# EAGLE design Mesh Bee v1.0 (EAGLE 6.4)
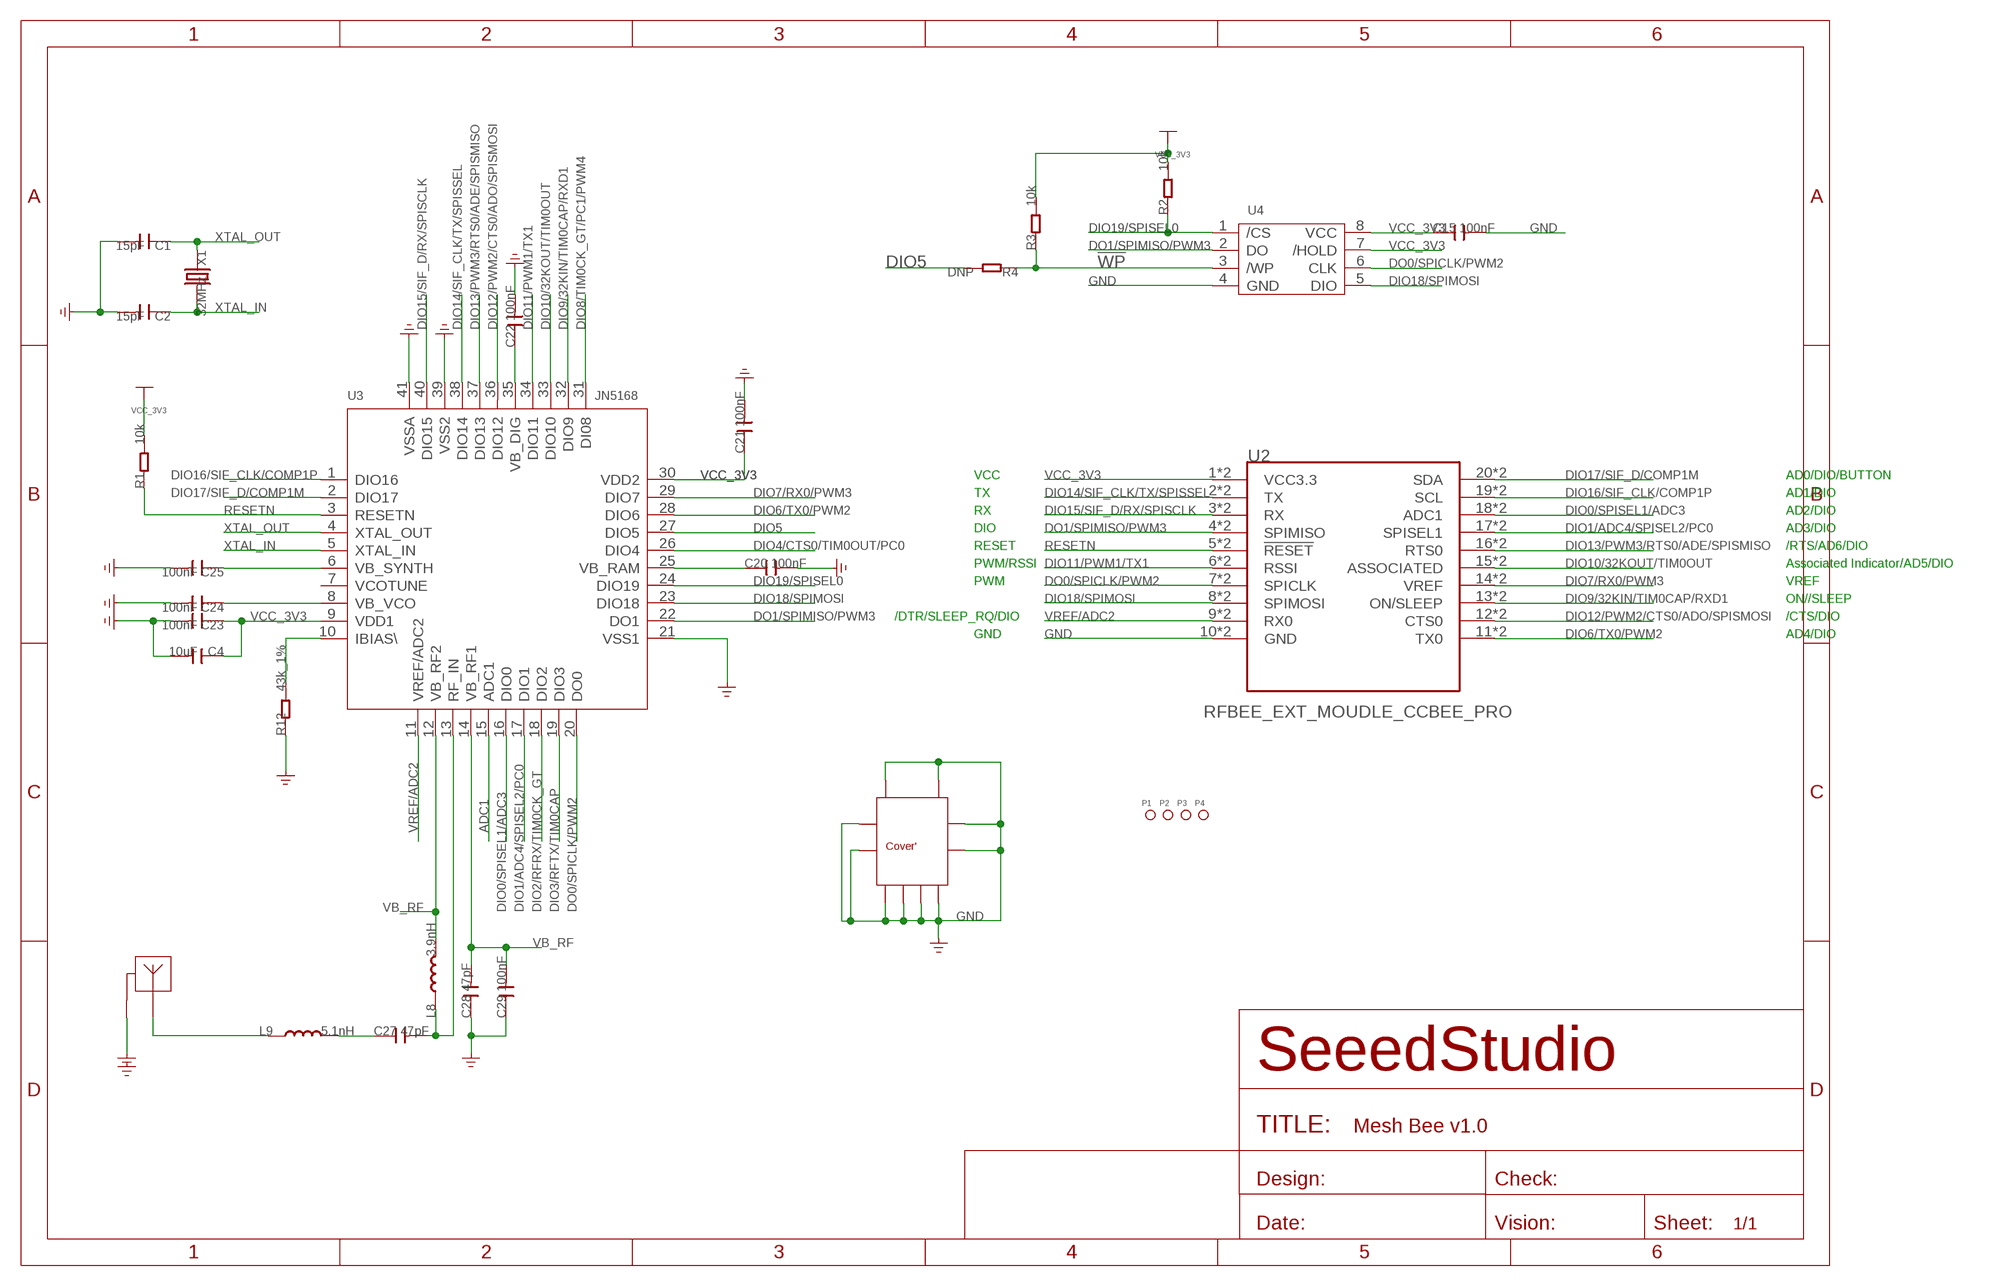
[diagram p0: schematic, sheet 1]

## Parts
ANT1  2.4G-ANT  [2.4G-ANT]
C1  15pF  C-0402  [C0402]
C2  15pF  C-0402  [C0402]
C4  10uF  C-0603  [C0603]
C15  100nF  C-0402  [C0402]
C20  100nF  C-0402  [C0402]
C21  100nF  C-0402  [C0402]
C22  100nF  C-0402  [C0402]
C23  100nF  C-0402  [C0402]
C24  100nF  C-0402  [C0402]
C25  100nF  C-0402  [C0402]
C27  47pF  C-0402  [C0402]
C28  47pF  C-0402  [C0402]
C29  100nF  C-0402  [C0402]
L8  3.9nH  L'0402'  [L0402]
L9  5.1nH  L'0402'  [L0402]
P1  PAD-MARK  [ROUND-MARK-1.0]
P2  PAD-MARK  [ROUND-MARK-1.0]
P3  PAD-MARK  [ROUND-MARK-1.0]
P4  PAD-MARK  [ROUND-MARK-1.0]
R1  10k  R-0402  [R0402]
R2  10k  R-0402  [R0402]
R3  10k  R-0402  [R0402]
R4  DNP  R-0402  [R0402]
R12  43k_1%  R-0402  [R0402]
U1  TEMPLATE_SHIELDING-COVER  [TEMPLATE_SHIELDING-COVER-20.6X18.5]
U2  RFBEE_EXT_MOUDLE_CCBEE_PRO  [RFBEE_EXT_MOUDLE_CCBEE-PRO]
U3  JN5168  [HVQFN40]
U4  W25X80  [WSON8]
X1  32MHz  CRYSTAL'3225'  [4P-SMD-3.2X2.5]

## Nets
!WP: R3.1 R4.1 U4.3(/WP)
ADC1: U3.15(ADC1)
DIO0/SPISEL1/ADC3: U2.18(ADC1) U2.P18(ADC1) U3.16(DIO0)
DIO1/ADC4/SPISEL2/PC0: U2.17(SPISEL1) U2.P17(SPISEL1) U3.17(DIO1)
DIO2/RFRX/TIM0CK_GT: U3.18(DIO2)
DIO3/RFTX/TIM0CAP: U3.19(DIO3)
DIO4/CTS0/TIM0OUT/PC0: U3.26(DIO4)
DIO5: R4.2 U3.27(DIO5)
DIO6/TX0/PWM2: U2.11(TX0) U2.P11(TX0) U3.28(DIO6)
DIO7/RX0/PWM3: U2.14(VREF) U2.P14(VREF) U3.29(DIO7)
DIO8/TIM0CK_GT/PC1/PWM4: U3.31(DI08)
DIO9/32KIN/TIM0CAP/RXD1: U2.13(ON/SLEEP) U2.P13(ON/SLEEP) U3.32(DIO9)
DIO10/32KOUT/TIM0OUT: U2.15(ASSOCIATED) U2.P15(ASSOCIATED) U3.33(DIO10)
DIO11/PWM1/TX1: U2.6(RSSI) U2.P6(RSSI) U3.34(DIO11)
DIO12/PWM2/CTS0/ADO/SPISMOSI: U2.12(CTS0) U2.P12(CTS0) U3.36(DIO12)
DIO13/PWM3/RTS0/ADE/SPISMISO: U2.16(RTS0) U2.P16(RTS0) U3.37(DIO13)
DIO14/SIF_CLK/TX/SPISSEL: U2.2(TX) U2.P2(TX) U3.38(DIO14)
DIO15/SIF_D/RX/SPISCLK: U2.3(RX) U2.P3(RX) U3.40(DIO15)
DIO16/SIF_CLK/COMP1P: U2.19(SCL) U2.P19(SCL) U3.1(DIO16)
DIO17/SIF_D/COMP1M: U2.20(SDA) U2.P20(SDA) U3.2(DIO17)
DIO18/SPIMOSI: U2.8(SPIMOSI) U2.P8(SPIMOSI) U3.23(DIO18) U4.5(DIO)
DIO19/SPISEL0: R2.1 U3.24(DIO19) U4.1(/CS)
DO0/SPICLK/PWM2: U2.7(SPICLK) U2.P7(SPICLK) U3.20(DO0) U4.6(CLK)
DO1/SPIMISO/PWM3: U2.4(SPIMISO) U2.P4(SPIMISO) U3.22(DO1) U4.2(DO)
GND: ANT1.1 C1.2 C2.2 C4.2 C15.2 C20.2 C21.2 C22.2 C23.2 C24.2 C25.2 C28.1 C29.1 R12.1 U1.P$1 U1.P$2 U1.P$3 U1.P$4 U1.P$5 U1.P$6 U1.P$7 U1.P$8 U1.P$9 U1.P$10 U2.10(GND) U2.P10(GND) U3.21(VSS1) U3.39(VSS2) U3.41(VSSA) U4.4(GND)
N$1: ANT1.2 L9.1
N$19: C20.1 U3.25(VB_RAM)
N$23: C22.1 U3.35(VB_DIG)
N$24: C25.1 U3.6(VB_SYNTH)
N$25: C24.1 U3.8(VB_VCO)
N$32: R12.2 U3.10(IBIAS\)
N$36: C27.2 L8.1 U3.13(RF_IN)
N$38: C27.1 L9.2
RESETN: R1.1 U2.5(!RESET) U2.P5(!RESET) U3.3(RESETN)
VB_RF: C28.2 C29.2 L8.2 U3.12(VB_RF2) U3.14(VB_RF1)
VCC_3V3: C4.1 C15.1 C21.1 C23.1 R1.2 R2.2 R3.2 U2.1(VCC3.3) U2.P1(VCC3.3) U3.9(VDD1) U3.30(VDD2) U4.7(/HOLD) U4.8(VCC)
VREF/ADC2: U2.9(RX0) U2.P9(RX0) U3.11(VREF/ADC2)
XTAL_IN: C2.1 U3.5(XTAL_IN) X1.4
XTAL_OUT: C1.1 U3.4(XTAL_OUT) X1.2
Unconnected: U3.7(VCOTUNE)

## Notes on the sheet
- VCC | AD0/DIO/BUTTON
- TX | AD1/DIO
- RX | AD2/DIO
- DIO | AD3/DIO
- RESET | /RTS/AD6/DIO
- PWM/RSSI | Associated Indicator/AD5/DIO
- PWM | VREF
- ON//SLEEP
- /DTR/SLEEP_RQ/DIO | /CTS/DIO
- GND | AD4/DIO

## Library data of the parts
ANT1 = template (quxiaohui quxiaohui 的冲突副本 2013-09-17):2.4G-ANT
C1 C2 C4 C15 C20-C25 C27-C29 = Discrete:C*: Ceramic Capacitors
L8 L9 = Discrete:L*
P1-P4 = Discrete:PAD-MARK; PARTNO: DNP
R1-R4 R12 = Discrete:R*
U1 = RFBee_-_REVA:TEMPLATE_SHIELDING-COVER
U2 = RFBee_-_REVA:RFBEE_EXT_MOUDLE_CCBEE
U3 = IC:JN5168: IEEE802.15.4 Wireless Microcontroller
U4 = template:W25X80: 1M-BIT,2M-BIT,4M-BIT AND 8M-BIT SERIAL FLASH MEMORY WITH 4KB SECTORS AND DUAL OUTPUT SPI
X1 = Discrete:CRYSTAL*: CRYSTAL

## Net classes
0 default: width 0.152 mm, drill 0.305 mm, clearance 0.152 mm

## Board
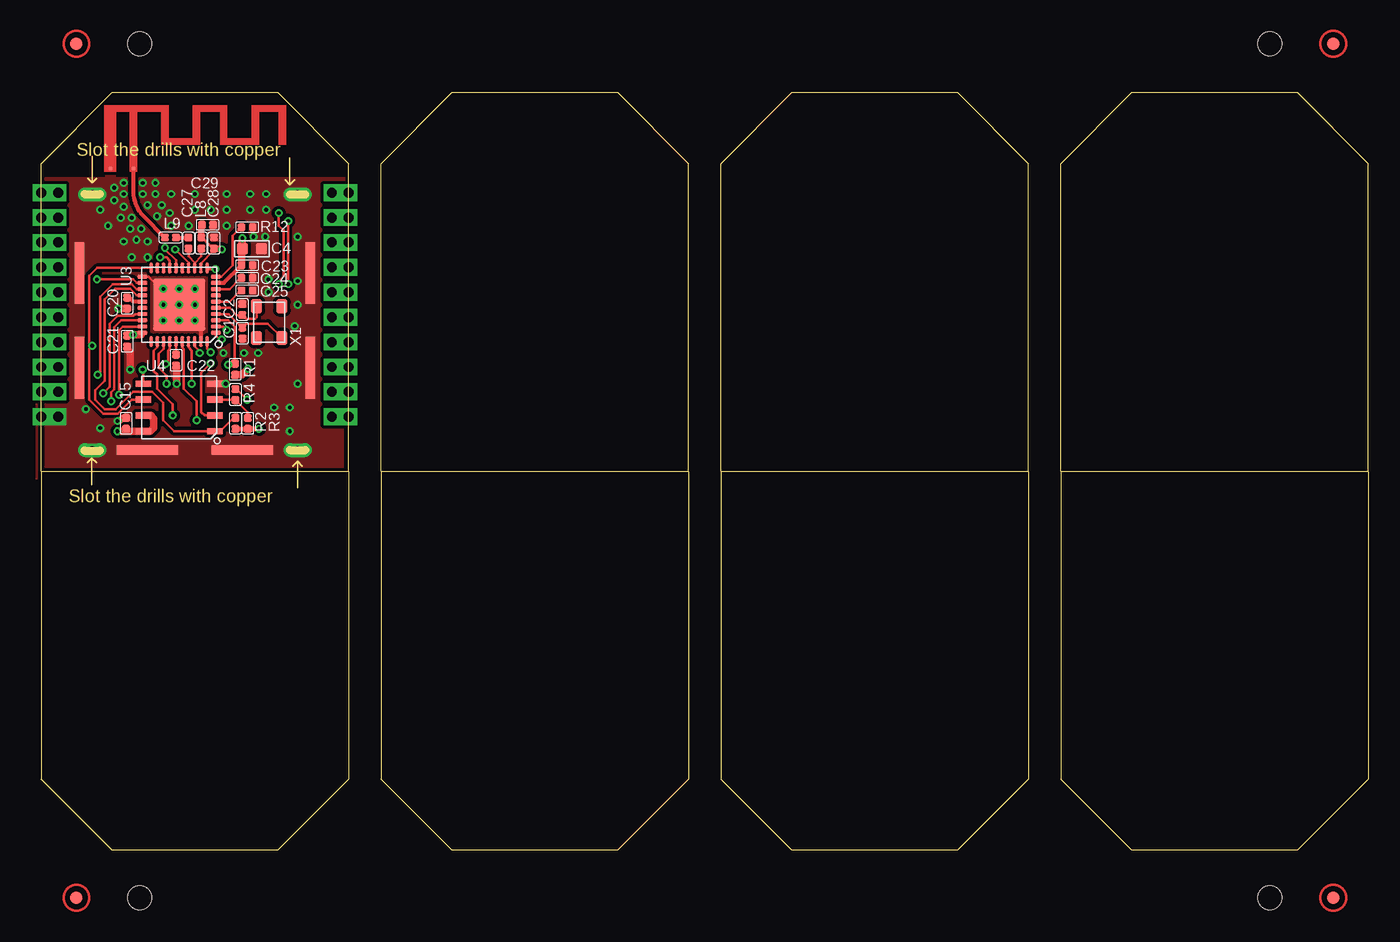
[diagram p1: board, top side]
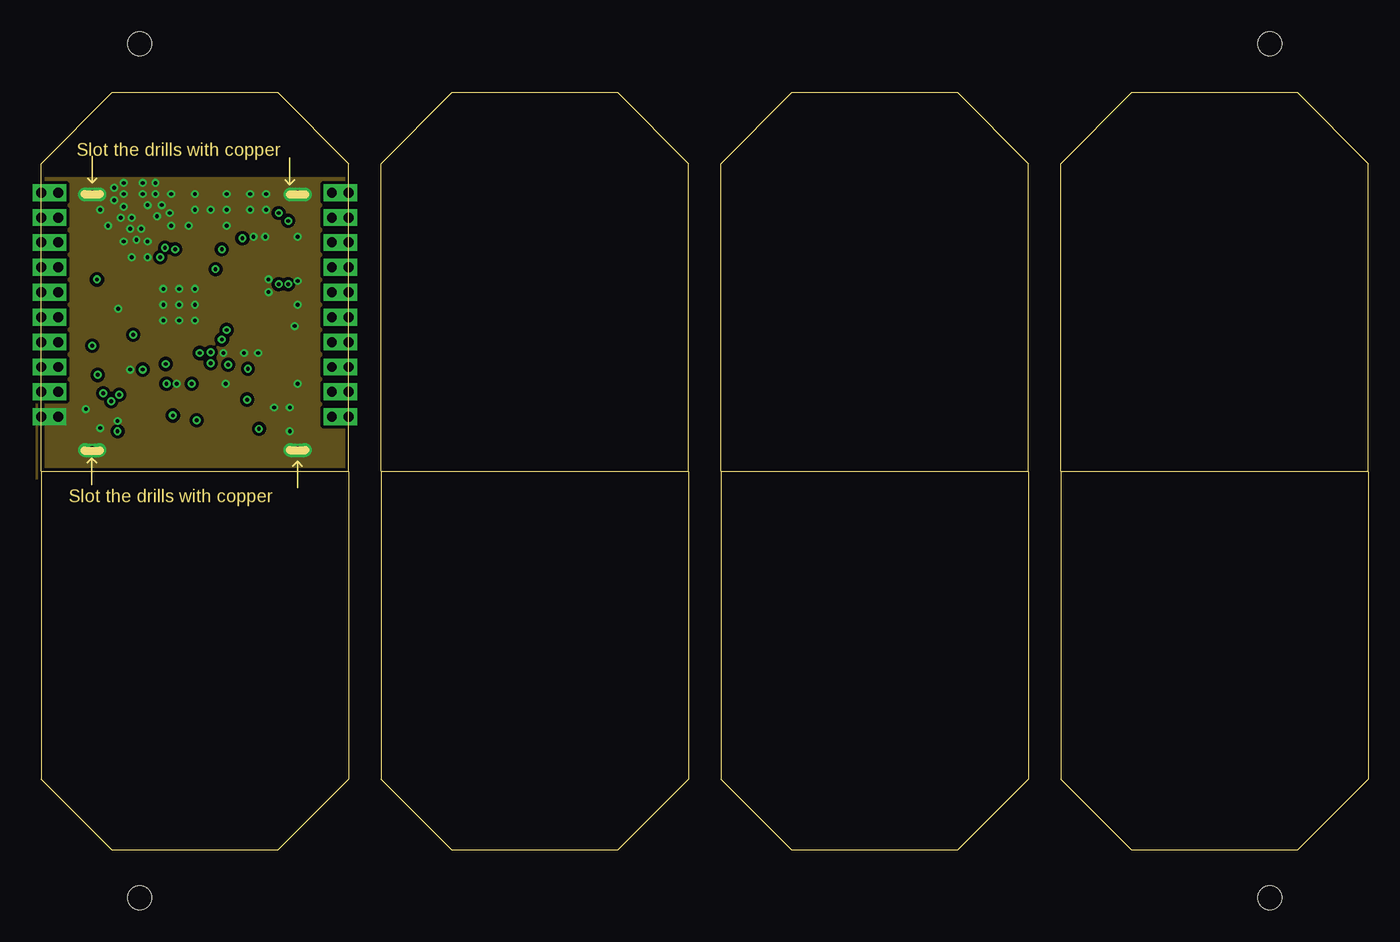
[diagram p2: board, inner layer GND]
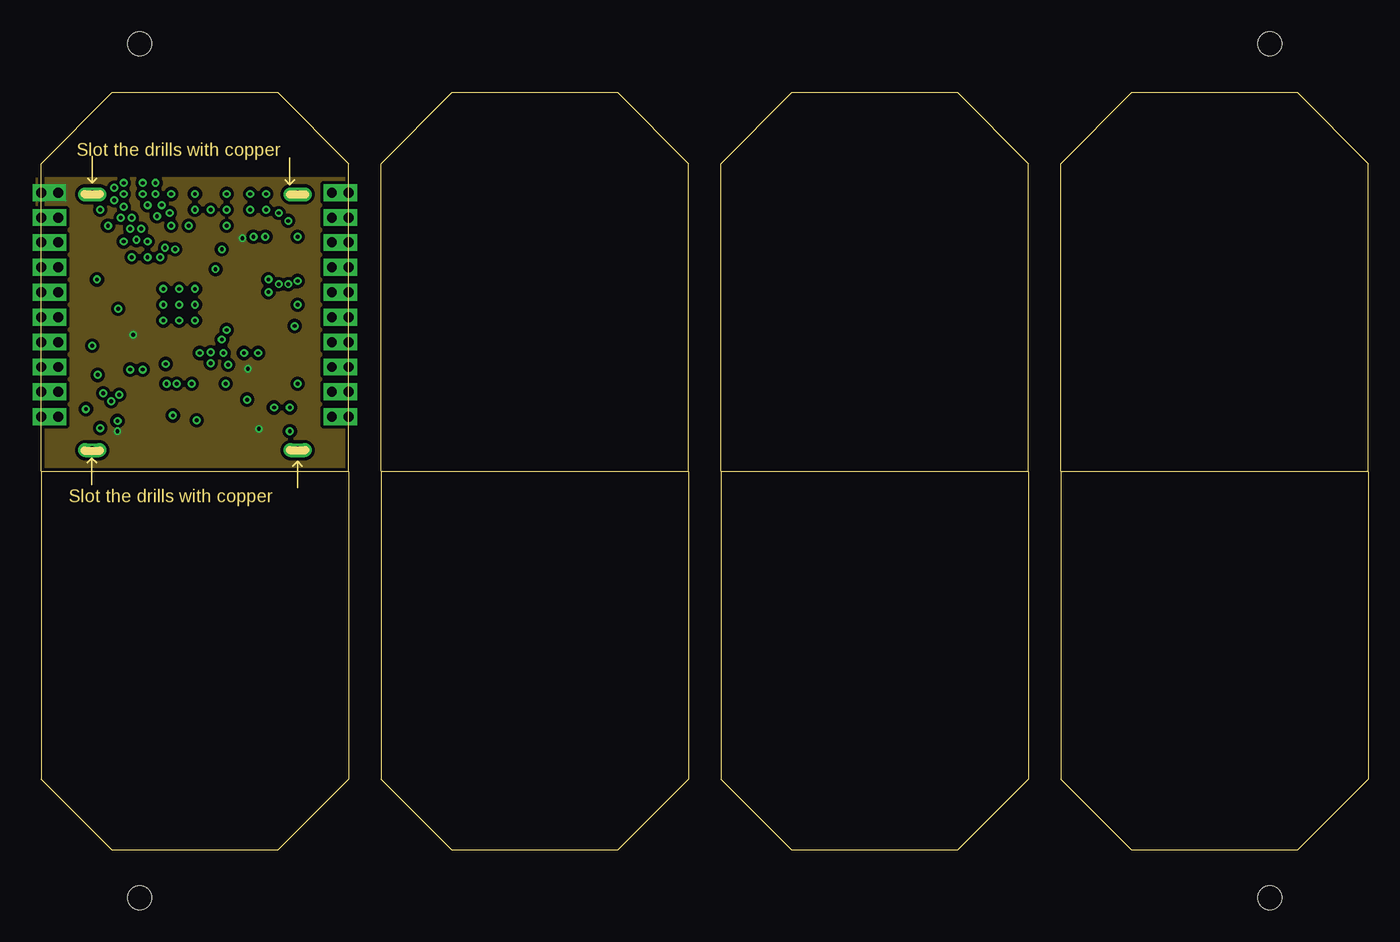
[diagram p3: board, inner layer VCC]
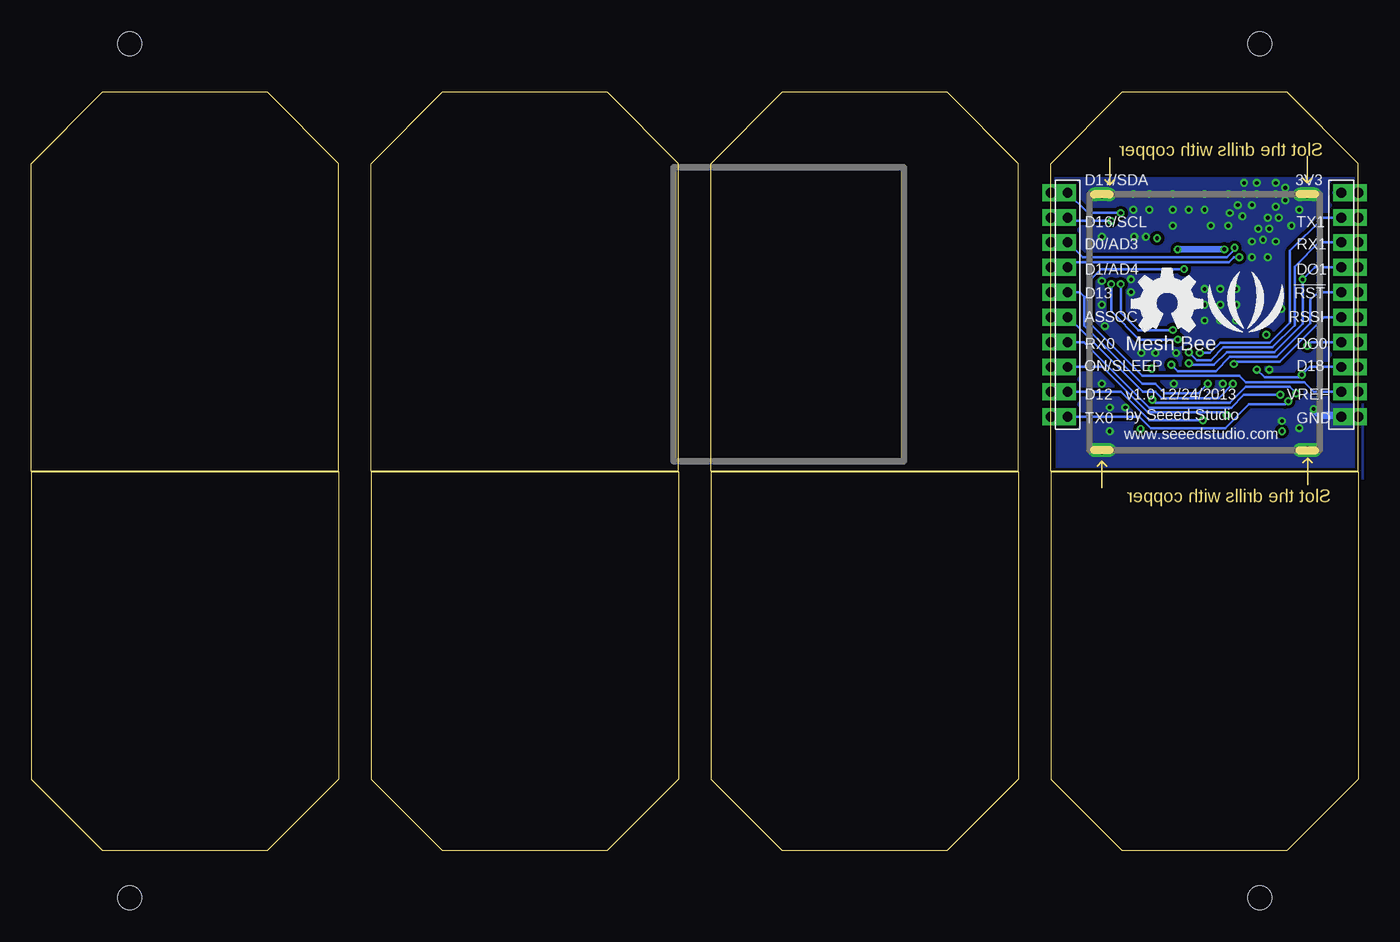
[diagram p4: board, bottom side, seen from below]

Size 106.61 x 60.87 mm. Coordinates in mm from the lower left corner, seen from the top.
Outline: 5.71,60.87 18.98,60.87 24.7,55.16 24.7,30.45 0,30.45 0,55.16 5.71,60.87
Outline: 18.98,0 5.71,0 0,5.71 0,30.43 24.7,30.43 24.7,5.71 18.98,0
Outline: 33.02,60.87 46.29,60.87 52.01,55.16 52.01,30.45 27.3,30.45 27.3,55.16 33.02,60.87
Outline: 46.29,0 33.02,0 27.3,5.71 27.3,30.43 52.01,30.43 52.01,5.71 46.29,0
Outline: 60.33,60.87 73.59,60.87 79.31,55.16 79.31,30.45 54.61,30.45 54.61,55.16 60.33,60.87
Outline: 73.59,0 60.33,0 54.61,5.71 54.61,30.43 79.31,30.43 79.31,5.71 73.59,0
Outline: 87.63,60.87 100.9,60.87 106.61,55.16 106.61,30.45 81.91,30.45 81.91,55.16 87.63,60.87
Outline: 100.9,0 87.63,0 81.91,5.71 81.91,30.43 106.61,30.43 106.61,5.71 100.9,0
Copper layers (1*2+15*16): Top 0.035mm / dielectric 0.2mm / GND 0.0175mm / dielectric 0.4mm / VCC 0.0175mm / dielectric 0.2mm / Bottom 0.035mm
Design rules "SeeedStudio_rule_no_angle_090911 *": minimum track width 6mil, minimum drill 12mil, track to track 6mil, track to pad 6mil, pad to pad 6mil, via to via 6mil, smd to smd 0mil, copper to edge 10mil, drill to drill 10mil, minimum pad ring 10mil, minimum via ring 6mil, stop-mask expansion 2mil, vias tented up to drill 100mil, thermal gap 10mil
Holes 1.91 mm at 7.9,64.78 98.71,64.78 7.9,-3.8 98.71,-3.8
tKeepout: area -4,47.9 to 30.3,61.1; area 29.4,47.3 to 63.7,60.5
tRestrict: area 24.6,29 to 24.6,34.2
bRestrict: area 24.6,29 to 24.6,34.2

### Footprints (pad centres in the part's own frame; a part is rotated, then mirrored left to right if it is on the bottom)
2.4G-ANT = smd 0.305 x 0.305: 1 0.457,0.254; 2 2.286,0.254
C0402 = smd 0.635 x 0.635: 1 -0.445,0; 2 0.445,0
C0603 = smd 0.889 x 0.889: 1 -0.762,0; 2 0.762,0
L0402 = smd 0.635 x 0.635: 1 -0.445,0; 2 0.445,0
ROUND-MARK-1.0 = smd 1.016 x 1.016: P$1 0,0
R0402 = smd 0.635 x 0.635: 1 -0.445,0; 2 0.445,0
TEMPLATE_SHIELDING-COVER-20.6X18.5 = drill 0.635 long: P$1 -8.255,-11.684; P$2 8.255,8.865; P$3 -8.255,8.865; P$4 8.255,-11.684 | smd 0.762 x 4.953: P$5 -9.271,2.54; P$6 -9.271,-5.055; P$7 9.271,2.54; P$8 9.271,-5.055 | smd 4.953 x 0.762: P$9 -3.81,-11.684; P$10 3.81,-11.684
RFBEE_EXT_MOUDLE_CCBEE-PRO = drill 0.8 pad 1.35 square: 1 -11,9; 2 -11,7; 3 -11,5; 4 -11,3; 5 -11,1; 6 -11,-1; 7 -11,-3; 8 -11,-5; 9 -11,-7; 10 -11,-9; 11 11,-9; 12 11,-7; 13 11,-5; 14 11,-3; 15 11,-1; 16 11,1; 17 11,3; 18 11,5; 19 11,7; 20 11,9; P1 -12.35,9; P2 -12.35,7; P3 -12.35,5; P4 -12.35,3; P5 -12.35,1; P6 -12.35,-1; P7 -12.35,-3; P8 -12.35,-5; P9 -12.35,-7; P10 -12.35,-9; P11 12.35,-9; P12 12.35,-7; P13 12.35,-5; P14 12.35,-3; P15 12.35,-1; P16 12.35,1; P17 12.35,3; P18 12.35,5; P19 12.35,7; P20 12.35,9
HVQFN40 = smd 0.8 x 0.3: 1 -2.95,2.25; 2 -2.95,1.75; 3 -2.95,1.25; 4 -2.95,0.75; 5 -2.95,0.25; 6 -2.95,-0.25; 7 -2.95,-0.75; 8 -2.95,-1.25; 9 -2.95,-1.75; 10 -2.95,-2.25; 21 2.95,-2.25; 22 2.95,-1.75; 23 2.95,-1.25; 24 2.95,-0.75; 25 2.95,-0.25; 26 2.95,0.25; 27 2.95,0.75; 28 2.95,1.25; 29 2.95,1.75; 30 2.95,2.25 | smd 0.3 x 0.8: 11 -2.25,-2.95; 12 -1.75,-2.95; 13 -1.25,-2.95; 14 -0.75,-2.95; 15 -0.25,-2.95; 16 0.25,-2.95; 17 0.75,-2.95; 18 1.25,-2.95; 19 1.75,-2.95; 20 2.25,-2.95; 31 2.25,2.95; 32 1.75,2.95; 33 1.25,2.95; 34 0.75,2.95; 35 0.25,2.95; 36 -0.25,2.95; 37 -0.75,2.95; 38 -1.25,2.95; 39 -1.75,2.95; 40 -2.25,2.95 | smd 4.2 x 4.2: 41 0,0
WSON8 = smd 0.5 x 1.25: 1 -1.905,-2.875; 2 -0.635,-2.875; 3 0.635,-2.875; 4 1.905,-2.875; 5 1.905,2.875; 6 0.635,2.875; 7 -0.635,2.875; 8 -1.905,2.875
4P-SMD-3.2X2.5 = smd 1.143 x 0.889: 1 -1.27,1.016; 2 -1.27,-1.016; 3 1.27,-1.016; 4 1.27,1.016

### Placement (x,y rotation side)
ANT1  5.11,54.49 0 top
C1  16.16,41.54 270 top
C2  16.16,43.44 90 top
C4  16.92,48.32 0 top
C15  6.81,34.3 90 top
C20  6.89,43.95 270 top
C21  6.89,40.9 270 top
C22  10.83,39.38 270 top
C23  16.54,47 0 top
C24  16.54,45.98 0 top
C25  16.54,44.96 0 top
C27  11.84,48.77 270 top
C28  13.87,48.77 270 top
C29  13.37,50.24 180 top
L8  12.86,48.77 90 top
L9  10.38,49.22 0 top
P1  not placed on the board
P2  not placed on the board
P3  not placed on the board
P4  not placed on the board
R1  15.58,38.64 270 top
R2  15.6,34.3 270 top
R3  16.59,34.3 270 top
R4  15.6,36.61 90 top
R12  16.54,50.04 180 top
U1  12.35,43.82 0 top
U2  12.35,43.82 0 top
U3  11.08,43.82 180 top
U4  11.08,35.57 90 top
U$16  [OSHW_FILLX200_NOTEXT]  18.19,41.66 0 bottom
U$17  [LOGO_SILK]  9.05,43.31 0 bottom
X1  18.32,42.42 90 top

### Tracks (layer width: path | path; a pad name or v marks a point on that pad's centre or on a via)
!WP
  Top 0.203: R3.1 16.59,35.17 R4.1 15.56,36.2 U4.3
DIO0/SPISEL1/ADC3  (via drill 0.3)
  Top 0.203: U3.16 10.83,47.37 9.94,48.27 v9.94,48.39
  Bottom 0.203: U2.18 23.32,48.82 22.13,47.63 10.57,47.63 9.94,48.27 v9.94,48.39
  Bottom 0.813: U2.18 U2.P18
DIO1/ADC4/SPISEL2/PC0  (via drill 0.3)
  Top 0.203: U3.17 10.33,47.37 10.06,47.63 v9.56,47.63
  Bottom 0.203: v9.56,47.63 10,47.63 10.38,47.25 22.92,47.25 U2.17
  Bottom 0.813: U2.17 U2.P17
DIO5  (via drill 0.3 pad 0.64)
  Top 0.203: U3.27 7.54,43.07 7.4,42.93 6.13,42.93 5.49,42.3 5.49,37.22 v4.98,36.71 | R4.2 15.69,37.05 v16.54,36.2
  Bottom 0.203: v4.98,36.71 5.49,37.22 9.05,37.22 10.32,35.95 16.29,35.95 v16.54,36.2
DIO6/TX0/PWM2  (via drill 0.3 pad 0.64)
  Top 0.203: U3.28 6.43,42.57 5.87,42.02 5.87,37.03 5.62,36.77 v5.62,36.07
  Bottom 0.203: v5.62,36.07 5.87,35.82 8.79,35.82 10.7,33.92 16.67,33.92 17.57,34.82 U2.11
  Bottom 0.813: U2.11 U2.P11
DIO7/RX0/PWM3  (via drill 0.3 pad 0.64)
  Top 0.203: U3.29 6.54,42.07 6.25,41.79 v6.25,36.58
  Bottom 0.203: v6.25,36.58 9.18,36.58 10.19,35.57 16.8,35.57 22.05,40.82 U2.14
  Bottom 0.813: U2.14 U2.P14
DIO9/32KIN/TIM0CAP/RXD1  (via drill 0.3 pad 0.64)
  Top 0.203: U3.32 9.33,40.42 9.05,40.14 9.05,38.49 9.3,38.23 9.3,37.09 10.57,35.82 v10.57,34.93
  Bottom 0.203: v10.57,34.93 10.83,35.19 16.92,35.19 20.56,38.82 U2.13
  Bottom 0.813: U2.13 U2.P13
DIO10/32KOUT/TIM0OUT  (via drill 0.3 pad 0.64)
  Top 0.203: U3.33 9.83,40.29 9.43,39.88 9.43,38.74 10.06,38.11 v10.06,37.47
  Bottom 0.203: U2.15 23.29,42.82 17.3,36.84 16.29,36.84 15.78,36.33 11.21,36.33 v10.06,37.47
  Bottom 0.813: U2.15 U2.P15
DIO11/PWM1/TX1  (via drill 0.3 pad 0.64)
  Top 0.203: U3.34 10.33,40.28 10.19,40.14 10.19,39.25 v10,39.06
  Bottom 0.203: U2.6 2.75,42.82 6.32,39.25 9.81,39.25 v10,39.06
  Bottom 0.813: U2.6 U2.P6
DIO12/PWM2/CTS0/ADO/SPISMOSI  (via drill 0.3 pad 0.64)
  Top 0.203: U3.36 11.33,40.4 11.46,40.27 11.46,37.09 12.48,36.07 v12.48,34.55
  Bottom 0.203: v12.48,34.55 16.8,34.55 19.07,36.82 U2.12
  Bottom 0.813: U2.12 U2.P12
DIO13/PWM3/RTS0/ADE/SPISMISO  (via drill 0.3 pad 0.64)
  Top 0.203: U3.37 11.83,40.4 12.1,40.14 v12.1,37.47
  Bottom 0.203: U2.16 22.37,44.82 22,44.46 22,42.14 17.33,37.47 16.29,37.47 15.52,36.71 12.86,36.71 v12.1,37.47
  Bottom 0.813: U2.16 U2.P16
DIO14/SIF_CLK/TX/SPISSEL  (via drill 0.3 pad 0.64)
  Top 0.203: U3.38 12.35,40.85 12.35,40.46 12.73,40.07 v12.73,39.95
  Bottom 0.203: U2.2 2.81,50.82 5.49,48.14 5.49,42.39 7.11,40.77 11.08,40.77 11.9,39.95 v12.73,39.95
  Bottom 0.813: U2.2 U2.P2
DIO15/SIF_D/RX/SPISCLK  (via drill 0.3 pad 0.64)
  Top 0.203: v13.62,40.01 13.33,40.3 U3.40
  Bottom 0.203: U2.3 3.16,48.82 5.11,46.87 5.11,42.18 6.9,40.39 10.83,40.39 11.84,39.38 12.98,39.38 v13.62,40.01
  Bottom 0.813: U2.3 U2.P3
DIO16/SIF_CLK/COMP1P  (via drill 0.3, 0.3 pad 0.64)
  Top 0.203: U3.1 14.03,41.38 14.38,41.03 v14.51,41.03 | v19.84,45.47 v19.84,50.55
  Bottom 0.203: v14.51,41.03 17.58,41.03 19.84,43.29 v19.84,45.47 | v19.84,50.55 23.08,50.55 U2.19
  Bottom 0.813: U2.19 U2.P19
DIO17/SIF_D/COMP1M  (via drill 0.3, 0.3 pad 0.64)
  Top 0.203: v19.08,51.19 19.08,50.17 19.46,49.79 19.46,46.11 19.08,45.73 v19.08,45.47 | U3.2 14.61,42.07 v14.89,41.79
  Bottom 0.203: v19.08,51.19 21.72,51.19 U2.20 | v19.08,45.47 19.08,43.19 17.68,41.79 v14.89,41.79
  Bottom 0.813: U2.20 U2.P20
DIO18/SPIMOSI  (via drill 0.3 pad 0.64)
  Top 0.203: U4.5 8.21,38.57 v8.16,38.61 | U3.23 7.67,45.07 7.27,45.47 5.75,45.47 4.73,44.46 4.73,38.38 v4.54,38.19
  Bottom 0.203: v8.16,38.61 7.52,37.98 4.75,37.98 v4.54,38.19 3.9,38.82 U2.8
  Bottom 0.813: U2.8 U2.P8
DIO19/SPISEL0
  Top 0.203: U3.24 7.66,44.57 7.14,45.09 5.92,45.09 5.11,44.28 5.11,37.73 4.35,36.96 4.35,36.2 5.11,35.44 6,35.44 7.4,36.84 8.92,36.84 9.81,35.95 9.81,34.55 10.7,33.66 U4.1 14.38,33.66 15.4,34.68 15.54,34.68 R2.1
DO0/SPICLK/PWM2  (via drill 0.3 pad 0.64)
  Top 0.203: U3.20 4.5,46.77 3.86,46.13 3.86,40.75 v4.09,40.52 3.86,40.28 3.86,36.19 4.98,35.06 6.13,35.06 7.27,36.2 U4.6
  Bottom 0.203: U2.7 3.79,40.82 v4.09,40.52
  Bottom 0.813: U2.7 U2.P7
DO1/SPIMISO/PWM3  (via drill 0.3 pad 0.64)
  Top 0.203: 8.29,45.6 8.16,45.6 U3.22 7.68,45.57 7.4,45.85 v4.48,45.85 | U4.2 13.11,34.93 12.85,35.2 12.85,38.35 v13.62,39.12
  Bottom 0.203: U2.4 3.51,46.82 v4.48,45.85 4.48,42.28 6.74,40.01 10.57,40.01 11.59,39 13.49,39 v13.62,39.12
  Bottom 0.813: U2.4 U2.P4
GND  (via drill 0.3 pad 0.64)
  Top 0.203: U3.21 8.64,46.07 9.56,45.15 9.75,45.15 v9.81,45.09
  Top 0.305: 13.87,50.17 C29.1
  Top 0.33: 10.19,44.58 10.32,44.58 U3.41 12.83,42.07 U3.39
  Top 0.508: 6.25,34.49 v6.13,34.49 6.32,34.49 6.63,34.8 6.89,34.8
  Top 0.61: C20.2 v6.19,43.5 | v10.89,37.47 10.89,38.87 C22.2 | C21.2 6.89,40.27 7.14,40.01 v7.14,38.61 | U4.4 v14.83,37.47
  Bottom 0.61: 1.46,34.93 3.08,34.93 v3.59,35.44
  Bottom 0.813: 1.46,34.93 U2.10 U2.P10
  other vias: 8.54,47.63 18.26,44.84 18.26,45.85 18,49.28 20.61,43.82 20.35,42.11 14.64,39.95 16.29,39.95 17.43,39.95 7.27,47.63 8.54,48.9 8.03,49.92 7.27,50.81 6.63,51.7 6.63,52.71 6.63,53.6 8.16,53.6 8.16,52.71 8.54,51.82 9.3,50.93 10.45,50.17 11.84,50.17 9.68,51.82 12.35,51.44 14.89,51.44 14.89,50.17 13.62,51.44 9.18,53.6 9.18,52.71 12.35,52.71 14.89,52.71 16.8,52.71 16.8,51.44 18.06,52.71 18.06,51.44 20.61,45.73 20.61,49.28 17.05,49.28 6.38,50.81 7.14,49.92 5.87,53.22 7.65,49.03 19.97,33.66 19.97,35.57 18.7,35.57 20.61,37.47 4.73,33.92 11.08,43.82 12.35,45.09 11.08,45.09 9.81,43.82 12.35,43.82 12.35,42.55 11.08,42.55 9.81,42.55 10.32,51.19 10.45,52.71 5.87,52.2 6.63,48.9 5.36,50.17 4.73,51.44
  pour Top (isolate 0.254, no thermals): 5.92,54.62 5.19,54.62 5.19,53.88 5.92,53.88
  pour GND (isolate 0.254, no thermals): -0.35,53.98 25.05,53.98 25.05,29.85 -0.35,29.85
  pour Bottom (isolate 0.254, no thermals): -0.35,53.98 25.05,53.98 25.05,29.85 -0.35,29.85
  pour Top (isolate 0.254, no thermals): -0.35,53.98 25.05,53.98 25.05,29.85 -0.35,29.85
N$1
  Top 0.33: ANT1.2 7.4,52.88 arc45 8.19,50.97 L9.1
N$19
  Top 0.305: U3.25 7.4,44.07 7.14,44.33 6.95,44.33 C20.1
N$23
  Top 0.203: U3.35 C22.1
N$24
  Top 0.203: U3.6 15.14,44.07 16.03,44.96 C25.1
N$25
  Top 0.203: U3.8 15.12,45.07 16.03,45.98 C24.1
N$32
  Top 0.203: U3.10 14.47,46.07 15.4,47 15.4,49.35 R12.2
N$36
  Top 0.203: U3.13 12.33,47.17 | 12.33,47.17 12.86,47.69 L8.1 | 12.33,47.17 12.33,47.21 11.84,47.69 C27.2
N$38
  Top 0.33: L9.2 C27.1
RESETN  (via drill 0.3 pad 0.64)
  Top 0.203: U3.3 15,42.57 15.52,42.04 15.52,39.14 R1.1 15.49,39 v15.02,39
  Bottom 0.203: v15.02,39 14.51,38.49 11.46,38.49 10.32,39.63 6.53,39.63 3.84,42.32 3.84,44.2 3.22,44.82 U2.5
  Bottom 0.813: U2.5 U2.P5
VB_RF  (via drill 0.3)
  Top 0.203: U3.12 12.83,47.16 13.81,48.14 13.81,48.27 | U3.14 11.83,47.2 v10.76,48.27 | 13.81,48.27 C28.2 | 13.81,48.27 13.75,48.27
  Top 0.254: L8.2 12.92,49.22 13.75,48.39 13.75,48.27
  Top 0.305: 12.86,50.17 C29.2
  Top 0.508: 12.86,50.17 L8.2 | C28.2 14.45,48.33 v14.51,48.27
  Bottom 0.508: v10.76,48.27 v14.51,48.27
VCC_3V3  (via drill 0.3, 0.3 pad 0.64)
  Top 0.305: U3.9 14.67,45.57 C23.1 | 8.03,41.41 8.03,41.47 U3.30
  Top 0.406: v17.49,33.85 R3.2 R2.2
  Top 0.61: v16.16,49.16 C4.1 16.1,48.25 C23.1 | C21.1 6.95,41.41 v7.4,41.41 8.03,41.41 | 7,33.66 U4.8 8.76,33.66 9.05,33.95 9.05,34.68 8.79,34.93 U4.7 | 7,33.66 C15.1 | v6.13,33.66 7,33.66 | R1.2 16.12,38.2 v16.61,38.68
  Bottom 0.61: U2.1 1.78,52.82
  Bottom 0.813: U2.1 U2.P1
  pour VCC (isolate 0.254, no thermals): -0.35,53.98 25.05,53.98 25.05,29.85 -0.35,29.85
VREF/ADC2  (via drill 0.3)
  Top 0.203: v14,46.68 13.42,46.68 U3.11
  Bottom 0.203: U2.9 3.57,36.82 4.35,37.6 9.05,37.6 9.56,38.11 17.35,38.11 21.49,42.25 21.49,45.85 20.67,46.68 v14,46.68
  Bottom 0.813: U2.9 U2.P9
XTAL_IN
  Top 0.203: X1.4 17.3,42.81 17.18,42.68 16.48,42.68 C2.1 15.71,43 15.14,43.57 U3.5
XTAL_OUT
  Top 0.203: U3.4 15.07,43.07 C1.1 | 16.1,41.92 C1.1 | X1.2 18.19,42.3 16.48,42.3 C1.1

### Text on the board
bPlace: 3V3 | D17/SDA | TX1 | D16/SCL | RX1 | D0/AD3 | DO1 | D1/AD4 | !RST | D13 | RSSI | ASSOC | DO0 | Mesh Bee | RX0 | D18 | ON/SLEEP | VREF | v1.0 12/24/2013 | D12 | by Seeed Studio | GND | TX0 | www.seeedstudio.com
